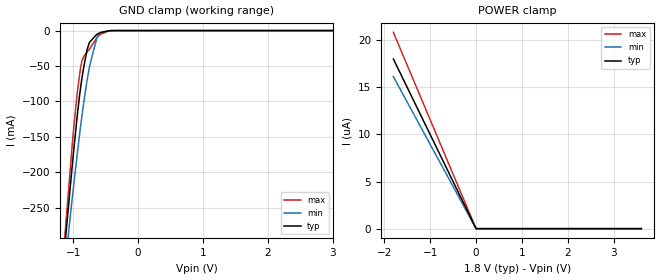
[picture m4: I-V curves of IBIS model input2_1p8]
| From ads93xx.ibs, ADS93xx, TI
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|   input2_1p8 Model
[Model]   input2_1p8
Model_type   Input
Vinl = 0.5
Vinh = 1.3
|   typ   min   max
C_comp   0.675pF   0.645pF   0.694pF
[Voltage Range]   1.8   1.65   1.95
[Temperature Range]   27   125   -40
[Power Clamp Reference]   1.8   1.65   1.95
[GND Clamp Reference]   0   0   0
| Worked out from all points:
|   GND clamp passes 1 mA (typ) near -0.49 V on its own axis
[GND Clamp]
|   Voltage   I(typ)   I(min)   I(max)
-1.8V     -1.014A    -945.4mA   -1.101A
-1.152V   -328.4mA   -355.7mA   -317.6mA
-1.022V   -198.9mA   -244.1mA   -170.1mA
-941.4mV  -124.4mA   -178mA     -92.2mA
-882mV    -78.34mA   -133mA     -50.39mA
-844.2mV  -55.73mA   -106.7mA   -38.1mA
-784.8mV  -26.73mA   -69.95mA   -30.23mA
-747mV    -16.48mA   -50.59mA   -25.77mA
-633.6mV  -5.342mA   -10.19mA   -10.19mA
-574.2mV  -2.667mA   -2.743mA   -4.977mA
-417.6mV  -118.9uA   -120.7uA   -150.7uA
3.6V      0A         0A         0A
[POWER Clamp]
|   Voltage   I(typ)   I(min)   I(max)
-1.8V     18uA       16.13uA    20.82uA
-1.8mV    13.92nA    12.82nA    16.64nA
9mV       0A         0A         0A
3.6V      0A         0A         0A
